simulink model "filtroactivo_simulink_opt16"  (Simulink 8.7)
settings: Solver=ode45  StartTime=0.0  StopTime=4  RelTol=1e-3
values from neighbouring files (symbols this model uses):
  C_LPF = 90e-6;5e-6;1e-6    [filtroactivo_simulink_opt16_default_values.m]    (also in filtroactivo_simulink_discrete_6_default_values.m; filtroactivo_LPF_C.m = 5.7e-06; filtroactivo_LPF_C_1.m = C; filtroactivo_LPF_C_2.m = 1.67e-05)
  Iload_dephase = 0*pi/180 * [1 0 0 0 0 0 0]    [filtroactivo_simulink_opt16_default_values.m]    (also in filtroactivo_simulink_discrete_6_default_values.m)
  Iload_freq = 50*[1 5 7 11 13 17 19]    [filtroactivo_simulink_opt16_default_values.m]    (also in filtroactivo_simulink_discrete_6_default_values.m)
  Iload_peak = 16*sqrt(2)/100*[100 10 10 10 10 0 0]    [filtroactivo_simulink_opt16_default_values.m]    (also in filtroactivo_simulink_discrete_6_default_values.m)
  Iload_sampletime = 1e-6    (= 1e-06)    [filtroactivo_simulink_opt16_default_values.m]    (also in filtroactivo_simulink_discrete_6_default_values.m)
  Iload_simetric = [-1 1 -1 1 -1 1 -1]    [filtroactivo_simulink_opt16_default_values.m]    (also in filtroactivo_simulink_discrete_6_default_values.m)
  kI_Ired_ref = 1e-3;1e-1    [filtroactivo_simulink_opt16_default_values.m]
  kP_Ired_ref = 1e-4;2.5e-4;1e-2    [filtroactivo_simulink_opt16_default_values.m]
  L_grid = 15e-6    (= 1.5e-05)    [filtroactivo_simulink_opt16_default_values.m]    (also in filtroactivo_simulink_discrete_6_default_values.m; filtroactivo_LPF_C_2.m)
  L_LPF = L    (= 0.004)    [filtroactivo_LPF_C.m]    (also in filtroactivo_LPF_C_1.m = L; filtroactivo_LPF_L.m = 0.001)
  period_SuSvSw = 1e-6    (= 1e-06)    [filtroactivo_simulink_opt16_default_values.m]    (also in filtroactivo_simulink_discrete_6_default_values.m)
  R_C_LPF = .1;.5    [filtroactivo_simulink_opt16_default_values.m]    (also in filtroactivo_simulink_discrete_6_default_values.m; filtroactivo_LPF_C.m = 0.5; filtroactivo_LPF_C_2.m = 0.5)
  R_grid = 0.02    [filtroactivo_simulink_opt16_default_values.m]    (also in filtroactivo_simulink_discrete_6_default_values.m; filtroactivo_LPF_C_2.m)
  R_L_LPF = .65;.125    [filtroactivo_simulink_opt16_default_values.m]    (also in filtroactivo_simulink_discrete_6_default_values.m; filtroactivo_LPF_C.m = 0.5)
  R_neutro_inverter_C_LPF = 1e-2;1;50;1e-2    [filtroactivo_simulink_opt16_default_values.m]    (also in filtroactivo_simulink_discrete_6_default_values.m)
  Vcc_desired = 900    [filtroactivo_simulink_opt16_default_values.m]    (also in filtroactivo_simulink_discrete_6_default_values.m)
  Vnet_dephase = 0*pi/180    (= 0)    [filtroactivo_simulink_opt16_default_values.m]    (also in filtroactivo_simulink_discrete_6_default_values.m)
  Vnet_freq = 50    [filtroactivo_simulink_opt16_default_values.m]    (also in filtroactivo_simulink_discrete_6_default_values.m)
  Vnet_peak = 566    [filtroactivo_simulink_opt16_default_values.m]    (also in filtroactivo_simulink_discrete_6_default_values.m)
libraries: powerlib x36

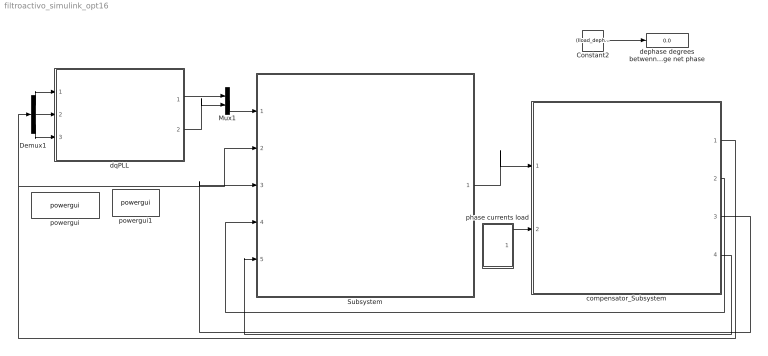
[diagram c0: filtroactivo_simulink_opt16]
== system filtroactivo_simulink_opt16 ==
  Constant2 : Constant  Value=(Iload_dephase(1) - Vnet_dephase(1))/(pi/180)
  Demux1 : Demux  Outputs=3
  Mux1 : Mux  Inputs=2
  Subsystem : Subsystem
  compensator_Subsystem : Subsystem
  dephase degrees betwenn: 1) current load phase 2) voltage net phase : Display
  dqPLL : ModelReference  ModelNameDialog=Park_method4_simulink_opt5_9_2.mdl  SimulationMode=Normal  ModelReferenceVersion=1.922
  phase currents load : Subsystem
  powergui : powerlib/powergui  Priority=1  SimulationMode=Discrete  SolverType=Tustin  SampleTime=500e-9  frequency=60  SPID=off  DisableSnubberDevices=off  DisableRonSwitches=off  DisableVfSwitches=off  SwTol=0  DisplayEquations=off  Interpol=off  ExternalGateDelay=off  methode=off  Ts=10  FunctionMessages=off  echomessages=off  HookPort=off  EnableUseOfTLC=off  x0status=blocks  frequencyindice=0  Pbase=100e6  ErrMax=1e-4  Iterations=50  UnitsV=kV  UnitsW=MW  buscounter=0  RestoreLinks=warning  ResistiveCurrentMeasurement=off  Frange=[0:2:500]  Ylog=off  Xlog=on  ShowGrid=off  save=off  variable=ZData  structure=ScopeData_compensator_Subsystem__Scope11  ZoomFFT=off  StartTime=0.5  cycles=5  DisplayStyle=1  fundamental=50  FreqAxis=on  MaxFrequency=20*50  frequencyindicesteady=1  RmsSteady=1  display=off
  powergui1 : powerlib/powergui  Priority=1  SimulationMode=Continuous  SolverType=Tustin/Backward Euler (TBE)  SampleTime=50e-6  frequency=60  SPID=off  DisableSnubberDevices=off  DisableRonSwitches=off  DisableVfSwitches=off  SwTol=0  DisplayEquations=off  Interpol=off  ExternalGateDelay=off  methode=off  Ts=10  FunctionMessages=off  echomessages=off  HookPort=off  EnableUseOfTLC=off  x0status=blocks  frequencyindice=60  Pbase=100e6  ErrMax=1e-4  Iterations=50  UnitsV=kV  UnitsW=MW  buscounter=0  RestoreLinks=warning  ResistiveCurrentMeasurement=off  Frange=[0:2:500]  Ylog=off  Xlog=on  ShowGrid=off  save=off  variable=ZData  structure=simout_I_phase_compensator_measured  ZoomFFT=off  StartTime=0.2  cycles=5  DisplayStyle=3  fundamental=50  FreqAxis=off  MaxFrequency=1000  frequencyindicesteady=1  RmsSteady=1  display=off
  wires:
  Subsystem/1(Iphase_compensator_reference) -> compensator_Subsystem/1(Iphase_compensator_reference)
  compensator_Subsystem/2(Vcc_ref-Vcc_measured) -> Subsystem/4(Vcc_ref-Vcc_measured)
  Constant2/1 -> dephase degrees betwenn: 1) current load phase 2) voltage net phase/1
  Mux1/1 -> Subsystem/1(Valpha&beta_phase_dqPLL)
  compensator_Subsystem/1(Vphase_net_measured) -> Demux1/1, Subsystem/2(Vphase_net_measured)
  compensator_Subsystem/3(Iphase_load_measured) -> Subsystem/3(I_phase_load_measured)
  compensator_Subsystem/4(Iphase_C_LPF_measured) -> Subsystem/5(Iphase_C_LPF_measured)
  phase currents load/1(Out1) -> compensator_Subsystem/2(Iphase_load_reference)
  Demux1/1 -> dqPLL/1
  Demux1/2 -> dqPLL/2
  Demux1/3 -> dqPLL/3
  dqPLL/1 -> Mux1/1
  dqPLL/2 -> Mux1/2

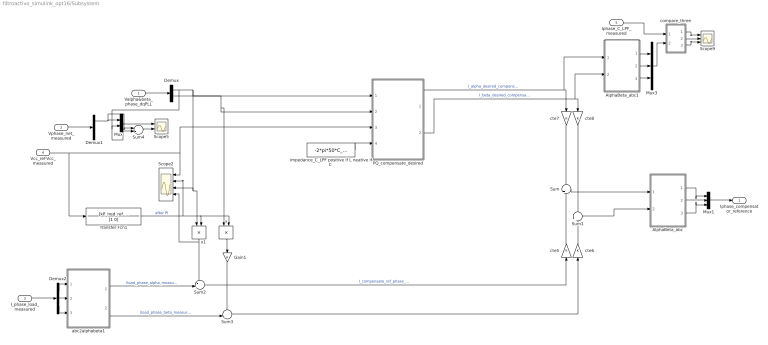
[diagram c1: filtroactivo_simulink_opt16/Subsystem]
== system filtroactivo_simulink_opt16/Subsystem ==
  Valpha&beta_phase_dqPLL : Inport
  Vphase_net_measured : Inport  Port=2
  I_phase_load_measured : Inport  Port=3
  Vcc_ref-Vcc_measured : Inport  Port=4
  Iphase_C_LPF_measured : Inport  Port=5
  AlphaBeta_abc : MATLAB Function  TreatAsAtomicUnit=on
  AlphaBeta_abc1 : MATLAB Function  TreatAsAtomicUnit=on
  Demux : Demux  Outputs=2
  Demux1 : Demux  Outputs=3
  Demux2 : Demux  Outputs=3
  Gain1 : Gain
  Mux : Mux  Inputs=2
  Mux1 : Mux  Inputs=3
  Mux3 : Mux  Inputs=3
  PQ_compensate_desired : Subsystem
  Scope2 : Scope  NumInputPorts=4
  Scope5 : Scope  NumInputPorts=2
  Scope9 : Scope  NumInputPorts=3
  Sum : Sum  Inputs=+|+
  Sum1 : Sum  Inputs=+|+
  Sum2 : Sum  Inputs=-+|
  Sum3 : Sum  Inputs=-+|
  Sum4 : Sum  Inputs=+-
  Transfer Fcn1 : TransferFcn  Numerator=[kP_Ired_ref kI_Ired_ref]  Denominator=[1 0]
  abc2alphabeta1 : MATLAB Function  TreatAsAtomicUnit=on
  compare_three : Subsystem
  cte{5..8} (4 alike) : Gain
  "impedance_C_LPF positive if L neative if C " : Constant  Value=-2*pi*50*C_LPF
  x : Product
  x1 : Product
  Iphase_compensator_reference : Outport  InitialOutput=0
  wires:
  AlphaBeta_abc/3(c) -> Mux1/3
  AlphaBeta_abc/2(b) -> Mux1/2
  AlphaBeta_abc/1(a) -> Mux1/1
  abc2alphabeta1/2(beta) -> Sum3/2  "Iload_phase_beta_measured"
  abc2alphabeta1/1(alpha) -> Sum2/2  "Iload_phase_alpha_measured"
  x/1 -> Gain1/1
  Sum/1 -> AlphaBeta_abc/1(alpha)
  Sum1/1 -> AlphaBeta_abc/2(beta)
  Sum2/1 -> cte5/1  "I_compensate_ref_phase_alpha_because_DVcc"
  Sum3/1 -> cte6/1
  cte7/1 -> Sum/1
  cte8/1 -> Sum1/1
  Vcc_ref-Vcc_measured/1 -> Transfer Fcn1/1, PQ_compensate_desired/3(Vcc_ref-Vcc_measured), Scope2/1
  Transfer Fcn1/1 -> Scope2/2, x1/2, x/2  "after PI"
  PQ_compensate_desired/2(Out2) -> AlphaBeta_abc1/2(beta), cte8/1  "I_beta_desired_compensate_PQ"
  PQ_compensate_desired/1(Out1) -> cte7/1, AlphaBeta_abc1/1(alpha)  "I_alpha_desired_compensate_PQ"
  Valpha&beta_phase_dqPLL/1 -> Demux/1
  Demux/1 -> Sum4/2, Mux/2, PQ_compensate_desired/1(Valpha), Scope2/3, x1/1
  Demux/2 -> x/1, PQ_compensate_desired/2(Vbeta)
  Vphase_net_measured/1 -> Demux1/1
  Demux1/1 -> Sum4/1, Mux/1
  Mux1/1 -> Iphase_compensator_reference/1
  Mux/1 -> Scope5/1
  Sum4/1 -> Scope5/2
  Demux2/2 -> abc2alphabeta1/2(b)
  Demux2/3 -> abc2alphabeta1/3(c)
  Demux2/1 -> abc2alphabeta1/1(a)
  cte5/1 -> Sum/2
  cte6/1 -> Sum1/2
  I_phase_load_measured/1 -> Demux2/1
  x1/1 -> Sum2/1, Scope2/4
  Gain1/1 -> Sum3/1
  "impedance_C_LPF positive if L neative if C "/1 -> PQ_compensate_desired/4(impedance_C_LPF)
  compare_three/1(Out1) -> Scope9/1
  compare_three/2(Out2) -> Scope9/2
  compare_three/3(Out3) -> Scope9/3
  Iphase_C_LPF_measured/1 -> compare_three/1(In1)
  AlphaBeta_abc1/1(a) -> Mux3/1
  AlphaBeta_abc1/2(b) -> Mux3/2
  AlphaBeta_abc1/3(c) -> Mux3/3
  Mux3/1 -> compare_three/2(In2)

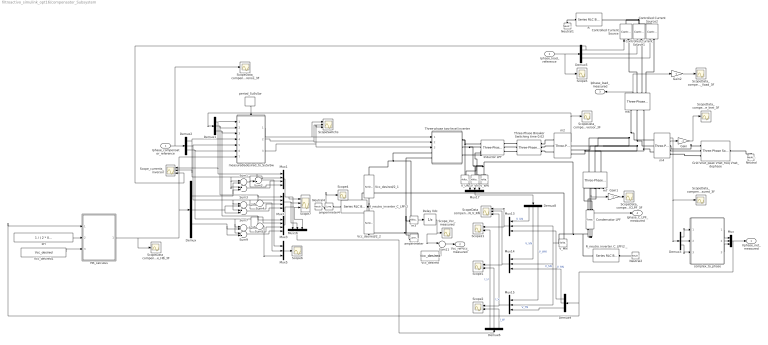
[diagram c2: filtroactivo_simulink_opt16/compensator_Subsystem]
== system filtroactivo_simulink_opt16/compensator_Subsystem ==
  Iphase_compensator_reference : Inport
  Iphase_load_reference : Inport  Port=2
  Condensator LPF : powerlib/Elements/Three-Phase Series RLC Branch  LConnTagsString=A|B|C  RConnTagsString=A|B|C  BranchType=RC  Resistance=R_C_LPF  Inductance=1e-3  Capacitance=C_LPF  Measurements=None
  Controlled Current Source : powerlib/Electrical Sources/Controlled Current Source  Initialize=off  Source_Type=AC  Amplitude=0  Phase=0  Frequency=0  Measurements=None
  Controlled Current Source1 : powerlib/Electrical Sources/Controlled Current Source  Initialize=off  Source_Type=AC  Amplitude=0  Phase=0  Frequency=0  Measurements=None
  Controlled Current Source2 : powerlib/Electrical Sources/Controlled Current Source  Initialize=off  Source_Type=AC  Amplitude=0  Phase=0  Frequency=0  Measurements=None
  Delay Vdc : UnitDelay  SampleTime=-1
  Demux{,1..3,5..6,8..9} (8 alike) : Demux  Outputs=3
  Gain : Gain  Gain=-1
  Gain1 : Gain  Gain=-1
  Gain2 : Gain  Gain=-1
  Grid Vnet_peak Vnet_freq Vnet_dephase : powerlib/Electrical Sources/Three-Phase Source  InternalConnection=Yn  VoltagePhases=off  Voltage=Vnet_peak/sqrt(2)  PhaseAngle=Vnet_dephase/pi*180  Voltage_phases=[25e3 25e3 25e3]/sqrt(3)  PhaseAngles_phases=[0 -120 +120]  Frequency=Vnet_freq  NonIdealSource=on  SpecifyImpedance=off  Resistance=R_grid  Inductance=L_grid  ShortCircuitLevel=100e6  BaseVoltage=25e3  XRratio=7  BusType=swing  Pref=0  Qref=0  Prefabc=[10e3, 10e3, 10e3]  Qrefabc=[0, 0, 0]  Qmin=-inf  Qmax=inf
  HB_calculus : MATLAB Function  TreatAsAtomicUnit=on
  Inductor LPF : powerlib/Elements/Three-Phase Series RLC Branch  LConnTagsString=A|B|C  RConnTagsString=A|B|C  BranchType=RL  Resistance=R_L_LPF  Inductance=L_LPF  Capacitance=1e-6  Measurements=None
  Mux{,5,13..17} (7 alike) : Mux  Inputs=3
  Mux1 : Mux
  Mux2 : Mux
  Mux3 : Mux
  Neutral : powerlib/Elements/Neutral  LConnTagsString=a  NodeNumber=1
  Neutral1 : powerlib/Elements/Neutral  LConnTagsString=a  NodeNumber=2
  Neutral2 : powerlib/Elements/Neutral  LConnTagsString=a  NodeNumber=2
  Neutral4 : powerlib/Elements/Neutral  LConnTagsString=a  NodeNumber=2
  R : powerlib/Elements/Series RLC Branch  LConnTagsString=__new0  RConnTagsString=__new0  BranchType=R  Resistance=1  Inductance=1e-3  SetiL0=off  InitialCurrent=0  Capacitance=1e-6  Setx0=off  InitialVoltage=0  Measurements=None
  R_neutro_inverter_C_LPF/2 : powerlib/Elements/Series RLC Branch  LConnTagsString=__new0  RConnTagsString=__new0  BranchType=R  Resistance=R_neutro_inverter_C_LPF/2  Inductance=1e-3  SetiL0=off  InitialCurrent=0  Capacitance=1e-6  Setx0=off  InitialVoltage=0  Measurements=None
  R_neutro_inverter_C_LPF/2 _ : powerlib/Elements/Series RLC Branch  LConnTagsString=__new0  RConnTagsString=__new0  BranchType=R  Resistance=R_neutro_inverter_C_LPF/2  Inductance=1e-3  SetiL0=off  InitialCurrent=0  Capacitance=1e-6  Setx0=off  InitialVoltage=0  Measurements=None
  Scope1 : Scope  NumInputPorts=2
  Scope2 : Scope  NumInputPorts=2
  Scope21 : Scope  NumInputPorts=2
  Scope4 : Scope
  Scope5 : Scope
  Scope6 : Scope
  Scope7 : Scope  NumInputPorts=3
  ScopeData_compensator_Subsystem__Scope_HB_3F : Scope
  ScopeData_compensator_Subsystem__Scope_ICLPF_3F : Scope
  ScopeData_compensator_Subsystem__Scope_Iinversor_3F : Scope
  ScopeData_compensator_Subsystem__Scope_Iinversorreference_3F : Scope
  ScopeData_compensator_Subsystem__Scope_Iload_3F : Scope
  ScopeData_compensator_Subsystem__Scope_Inet_3F : Scope
  ScopeData_compensator_Subsystem__Scope_V_UN_V_MN_V_RN : Scope  NumInputPorts=3
  ScopeData_compensator_Subsystem__Scope_Vnet_measured_3F : Scope
  ScopeSwitchs : Scope  NumInputPorts=3
  Scope_Vcc_measured : Scope
  Scope_currents_inversor : Scope  NumInputPorts=3
  Sum1 : Sum  Inputs=+-
  Sum11 : Sum  Inputs=|-+
  Sum2 : Sum  Inputs=-+|
  Sum3 : Sum
  Sum4 : Sum  Inputs=-+|
  Sum5 : Sum  Inputs=-+|
  Sum6 : Sum  Inputs=+-
  Sum7 : Sum
  Sum8 : Sum  Inputs=+-
  Sum9 : Sum
  Three-Phase Breaker Switching time 0.02 : powerlib/Elements/Three-Phase Breaker  InitialState=open  SwitchA=on  SwitchB=on  SwitchC=on  SwitchTimes=[0.020]  External=off  BreakerResistance=0.001  SnubberResistance=1e6  SnubberCapacitance=inf  Measurements=None
  Three-phase two-level inverter : Subsystem
  V_MN : powerlib/Measurements/Voltage Measurement  PhasorSimulation=off  OutputType=Complex  PSBequivalent=0
  V_UN : powerlib/Measurements/Voltage Measurement  PhasorSimulation=off  OutputType=Complex  PSBequivalent=0
  V_VN : powerlib/Measurements/Voltage Measurement  PhasorSimulation=off  OutputType=Complex  PSBequivalent=0
  V_WN : powerlib/Measurements/Voltage Measurement  PhasorSimulation=off  OutputType=Complex  PSBequivalent=0
  Vcc_desired : Constant  Value=Vcc_desired
  Vcc_desired/2_1 : powerlib/Elements/Series RLC Branch  LConnTagsString=__new0  RConnTagsString=__new0  BranchType=C  Resistance=0  Inductance=0  SetiL0=off  InitialCurrent=0  Capacitance=1e-2  Setx0=on  InitialVoltage=Vcc_desired/2  Measurements=None
  Vcc_desired/2_2 : powerlib/Elements/Series RLC Branch  LConnTagsString=__new0  RConnTagsString=__new0  BranchType=C  Resistance=0  Inductance=0  SetiL0=off  InitialCurrent=0  Capacitance=1e-2  Setx0=on  InitialVoltage=Vcc_desired/2  Measurements=None
  Vcc_desired1 : Constant  Value=Vcc_desired
  amperimeter : powerlib/Measurements/Current Measurement  PhasorSimulation=off  OutputType=Complex  PSBequivalent=0
  amperimeter4 : powerlib/Measurements/Current Measurement  PhasorSimulation=off  OutputType=Complex  PSBequivalent=0
  complex_to_phase : MATLAB Function  TreatAsAtomicUnit=on
  kH : Constant  Value=1 / ( 2 * 0.005 * 25e3 *Vcc_desired )
  m{2,4,6..7} (4 alike) : powerlib/Measurements/Three-Phase V-I Measurement  VoltageMeasurement=phase-to-phase  SetLabelV=off  LabelV=Vabc  Vpu=off  VpuLL=off  CurrentMeasurement=yes  SetLabelI=off  LabelI=Iabc  Ipu=off  Pbase=100e6  Vbase=500e3  OutputType=Complex  PhasorSimulation=off  PSBequivalent=0
  m3 : powerlib/Measurements/Voltage Measurement  PhasorSimulation=off  OutputType=Complex  PSBequivalent=0
  measured&desired_to_SuSvSw : Subsystem
  period_SuSvSw : DiscretePulseGenerator  PulseType=Time based  Period=period_SuSvSw  PulseWidth=50
  Vphase_net_measured : Outport
  Vcc_ref-Vcc_measured : Outport  Port=2
  Iphase_load_measured : Outport  Port=3
  Iphase_C_LPF_measured : Outport  Port=4
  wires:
  period_SuSvSw/1 -> measured&desired_to_SuSvSw/Trigger
  Demux2/1 -> measured&desired_to_SuSvSw/4(Iu*), Sum2/2, Mux1/2, Sum1/1, Sum3/1, Scope_currents_inversor/2
  Demux2/2 -> measured&desired_to_SuSvSw/5(Iv*), Sum7/1, Sum6/1, Mux2/2, Sum4/2
  Demux2/3 -> measured&desired_to_SuSvSw/6(Iw*), Sum9/1, Sum8/1, Mux3/2, Sum5/2
  Sum1/1 -> Mux1/4
  Sum3/1 -> Mux1/3
  Sum6/1 -> Mux2/3
  Sum8/1 -> Mux3/3
  Demux/1 -> Sum1/2, Sum3/2
  Demux/2 -> Sum6/2, Sum7/2
  Demux/3 -> Sum9/2, Sum8/2
  m3/1 -> Delay Vdc/1
  Delay Vdc/1 -> Sum11/1, Scope_Vcc_measured/1
  HB_calculus/1(HB) -> ScopeData_compensator_Subsystem__Scope_HB_3F/1, Demux/1, measured&desired_to_SuSvSw/7(H)
  m4/1 -> ScopeData_compensator_Subsystem__Scope_Vnet_measured_3F/1, Demux3/1
  m4/2 -> Gain/1
  Demux1/2 -> Sum4/1, Mux2/1, measured&desired_to_SuSvSw/2(Iv)
  Demux1/3 -> measured&desired_to_SuSvSw/3(Iw), Sum5/1, Mux3/1
  Demux1/1 -> Scope_currents_inversor/1, Sum2/1, Mux1/1, measured&desired_to_SuSvSw/1(Iu)
  Demux5/1 -> Scope_currents_inversor/3, Controlled Current Source/1
  Demux5/2 -> Controlled Current Source1/1
  Demux5/3 -> Controlled Current Source2/1
  m7/2 -> Gain1/1, Iphase_C_LPF_measured/1
  Iphase_load_reference/1 -> Scope5/1, Demux5/1
  m6/2 -> Gain2/1, Iphase_load_measured/1
  Mux5/1 -> Scope6/1
  Sum2/1 -> Mux5/1
  Sum4/1 -> Mux5/2
  Sum5/1 -> Mux5/3
  Sum7/1 -> Mux2/4
  Sum9/1 -> Mux3/4
  Gain/1 -> ScopeData_compensator_Subsystem__Scope_Inet_3F/1
  m2/2 -> ScopeData_compensator_Subsystem__Scope_Iinversor_3F/1, Demux1/1
  Sum11/1 -> Vcc_ref-Vcc_measured/1
  Vcc_desired/1 -> Sum11/2
  Demux3/2 -> complex_to_phase/2(Vst)
  Demux3/1 -> complex_to_phase/1(Vrs)
  Demux3/3 -> complex_to_phase/3(Vtr)
  complex_to_phase/2(Vs) -> Mux/2
  complex_to_phase/3(Vt) -> Mux/3
  complex_to_phase/1(Vr) -> Mux/1
  Iphase_compensator_reference/1 -> ScopeData_compensator_Subsystem__Scope_Iinversorreference_3F/1, Demux2/1
  amperimeter4/1 -> Scope4/1
  measured&desired_to_SuSvSw/3(Sw) -> Three-phase two-level inverter/3(Sc), ScopeSwitchs/3
  measured&desired_to_SuSvSw/2(Sv) -> ScopeSwitchs/2, Three-phase two-level inverter/2(Sb)
  measured&desired_to_SuSvSw/1(Su) -> ScopeSwitchs/1, Three-phase two-level inverter/1(Sa)
  Mux/1 -> Demux9/1, HB_calculus/1(Vfaseneutro), Vphase_net_measured/1
  kH/1 -> HB_calculus/2(Kh)
  Vcc_desired1/1 -> HB_calculus/3(Vcc_desired)
  Gain1/1 -> ScopeData_compensator_Subsystem__Scope_ICLPF_3F/1
  V_VN/1 -> Mux17/2
  V_WN/1 -> Mux17/3
  V_UN/1 -> Mux17/1
  Mux13/1 -> Scope21/1, ScopeData_compensator_Subsystem__Scope_V_UN_V_MN_V_RN/1
  Mux14/1 -> Scope1/1, ScopeData_compensator_Subsystem__Scope_V_UN_V_MN_V_RN/2
  V_MN/1 -> Mux15/2, Mux14/2, Mux13/2
  Demux8/1 -> Mux13/1  "V_UN"
  Demux8/2 -> Mux14/1  "V_VN"
  Demux8/3 -> Mux15/1  "V_WN"
  Demux9/1 -> Mux13/3  "V_RN"
  Demux9/2 -> Mux14/3  "V_SN"
  Demux9/3 -> Mux15/3  "V_TN"
  Mux15/1 -> Scope2/1, ScopeData_compensator_Subsystem__Scope_V_UN_V_MN_V_RN/3
  Mux17/1 -> Demux8/1
  Mux1/1 -> Mux16/1, Scope7/1
  Mux2/1 -> Mux16/2, Scope7/2
  Mux3/1 -> Mux16/3, Scope7/3
  Mux16/1 -> Demux6/1
  Demux6/1 -> Scope21/2  "I_U"
  Demux6/2 -> Scope1/2  "I_V"
  Demux6/3 -> Scope2/2  "I_W"
  Gain2/1 -> ScopeData_compensator_Subsystem__Scope_Iload_3F/1
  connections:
  Three-phase two-level inverter/RConn1 -- V_UN/LConn1 -- Inductor LPF/LConn1
  Three-phase two-level inverter/RConn2 -- V_VN/LConn1 -- Inductor LPF/LConn2
  Vcc_desired/2_2/RConn1 -- m3/LConn2 -- amperimeter/LConn1
  Three-phase two-level inverter/LConn1 -- Vcc_desired/2_1/LConn1 -- m3/LConn1
  m6/LConn1 -- m7/LConn1 -- m2/RConn1 -- m4/LConn1
  Controlled Current Source1/RConn1 -- R/RConn1 -- Controlled Current Source/RConn1 -- Controlled Current Source2/RConn1
  m6/LConn2 -- m7/LConn2 -- m2/RConn2 -- m4/LConn2
  m6/LConn3 -- m7/LConn3 -- m2/RConn3 -- m4/LConn3
  m6/RConn1 -- Controlled Current Source/LConn1
  Neutral1/LConn1 -- R/LConn1
  m4/RConn2 -- Grid Vnet_peak Vnet_freq Vnet_dephase/RConn2
  Grid Vnet_peak Vnet_freq Vnet_dephase/LConn1 -- Neutral/LConn1
  Condensator LPF/LConn1 -- m7/RConn1
  m4/RConn1 -- Grid Vnet_peak Vnet_freq Vnet_dephase/RConn1
  Condensator LPF/LConn3 -- m7/RConn3
  Three-Phase Breaker Switching time 0.02/RConn1 -- m2/LConn1
  Condensator LPF/LConn2 -- m7/RConn2
  m6/RConn2 -- Controlled Current Source1/LConn1
  amperimeter/RConn1 -- Three-phase two-level inverter/LConn2
  Three-Phase Breaker Switching time 0.02/RConn3 -- m2/LConn3
  Three-Phase Breaker Switching time 0.02/RConn2 -- m2/LConn2
  m6/RConn3 -- Controlled Current Source2/LConn1
  R_neutro_inverter_C_LPF/2 _/LConn1 -- Neutral2/LConn1
  Inductor LPF/LConn3 -- V_WN/LConn1 -- Three-phase two-level inverter/RConn3
  m4/RConn3 -- Grid Vnet_peak Vnet_freq Vnet_dephase/RConn3
  R_neutro_inverter_C_LPF/2/RConn1 -- V_MN/LConn1 -- Vcc_desired/2_1/RConn1 -- Vcc_desired/2_2/LConn1
  amperimeter4/LConn1 -- Neutral4/LConn1
  amperimeter4/RConn1 -- R_neutro_inverter_C_LPF/2/LConn1
  Inductor LPF/RConn1 -- Three-Phase Breaker Switching time 0.02/LConn1
  Inductor LPF/RConn2 -- Three-Phase Breaker Switching time 0.02/LConn2
  Inductor LPF/RConn3 -- Three-Phase Breaker Switching time 0.02/LConn3
  Condensator LPF/RConn1 -- V_VN/LConn2 -- V_UN/LConn2 -- V_WN/LConn2 -- V_MN/LConn2 -- R_neutro_inverter_C_LPF/2 _/RConn1 -- Condensator LPF/RConn3 -- Condensator LPF/RConn2

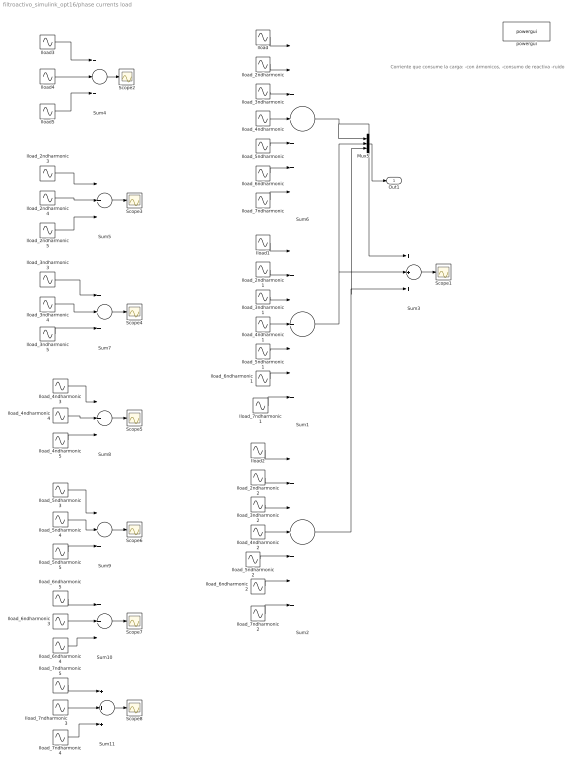
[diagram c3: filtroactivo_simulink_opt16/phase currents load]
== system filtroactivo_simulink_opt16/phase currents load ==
  note: Corriente que consume la carga: -con ármonicos, -consumo de reactiva -ruido
  Iload : Sin  Amplitude=Iload_peak(1)  Frequency=2*pi*Iload_freq(1)  Phase=Iload_dephase(1)  SampleTime=Iload_sampletime
  Iload1 : Sin  Amplitude=Iload_peak(1)  Frequency=2*pi*Iload_freq(1)  Phase=Iload_dephase(1) + 2*pi/3*Iload_simetric(1)  SampleTime=Iload_sampletime
  Iload2 : Sin  Amplitude=Iload_peak(1)  Frequency=2*pi*Iload_freq(1)  Phase=Iload_dephase(1) + 4*pi/3*Iload_simetric(1)  SampleTime=Iload_sampletime
  Iload3 : Sin  Amplitude=Iload_peak(1)  Frequency=2*pi*Iload_freq(1)  Phase=Iload_dephase(1)  SampleTime=Iload_sampletime
  Iload4 : Sin  Amplitude=Iload_peak(1)  Frequency=2*pi*Iload_freq(1)  Phase=Iload_dephase(1) + 2*pi/3*Iload_simetric(1)  SampleTime=Iload_sampletime
  Iload5 : Sin  Amplitude=Iload_peak(1)  Frequency=2*pi*Iload_freq(1)  Phase=Iload_dephase(1) + 4*pi/3*Iload_simetric(1)  SampleTime=Iload_sampletime
  Iload_2ndharmonic : Sin  Amplitude=Iload_peak(2)  Frequency=2*pi*Iload_freq(2)  Phase=Iload_dephase(2)  SampleTime=Iload_sampletime
  Iload_2ndharmonic1 : Sin  Amplitude=Iload_peak(2)  Frequency=2*pi*Iload_freq(2)  Phase=Iload_dephase(2) + 2*pi/3*Iload_simetric(2)  SampleTime=Iload_sampletime
  Iload_2ndharmonic2 : Sin  Amplitude=Iload_peak(2)  Frequency=2*pi*Iload_freq(2)  Phase=Iload_dephase(2) + 4*pi/3*Iload_simetric(2)  SampleTime=Iload_sampletime
  Iload_2ndharmonic3 : Sin  Amplitude=Iload_peak(2)  Frequency=2*pi*Iload_freq(2)  Phase=Iload_dephase(2)  SampleTime=Iload_sampletime
  Iload_2ndharmonic4 : Sin  Amplitude=Iload_peak(2)  Frequency=2*pi*Iload_freq(2)  Phase=Iload_dephase(2) + 2*pi/3*Iload_simetric(2)  SampleTime=Iload_sampletime
  Iload_2ndharmonic5 : Sin  Amplitude=Iload_peak(2)  Frequency=2*pi*Iload_freq(2)  Phase=Iload_dephase(2) + 4*pi/3*Iload_simetric(2)  SampleTime=Iload_sampletime
  Iload_3ndharmonic : Sin  Amplitude=Iload_peak(3)  Frequency=2*pi*Iload_freq(3)  Phase=Iload_dephase(3)  SampleTime=Iload_sampletime
  Iload_3ndharmonic1 : Sin  Amplitude=Iload_peak(3)  Frequency=2*pi*Iload_freq(3)  Phase=Iload_dephase(3) + 2*pi/3*Iload_simetric(3)  SampleTime=Iload_sampletime
  Iload_3ndharmonic2 : Sin  Amplitude=Iload_peak(3)  Frequency=2*pi*Iload_freq(3)  Phase=Iload_dephase(3) + 4*pi/3*Iload_simetric(3)  SampleTime=Iload_sampletime
  Iload_3ndharmonic3 : Sin  Amplitude=Iload_peak(3)  Frequency=2*pi*Iload_freq(3)  Phase=Iload_dephase(3)  SampleTime=Iload_sampletime
  Iload_3ndharmonic4 : Sin  Amplitude=Iload_peak(3)  Frequency=2*pi*Iload_freq(3)  Phase=Iload_dephase(3) + 2*pi/3*Iload_simetric(3)  SampleTime=Iload_sampletime
  Iload_3ndharmonic5 : Sin  Amplitude=Iload_peak(3)  Frequency=2*pi*Iload_freq(3)  Phase=Iload_dephase(3) + 4*pi/3*Iload_simetric(3)  SampleTime=Iload_sampletime
  Iload_4ndharmonic : Sin  Amplitude=Iload_peak(4)  Frequency=2*pi*Iload_freq(4)  Phase=Iload_dephase(4)  SampleTime=Iload_sampletime
  Iload_4ndharmonic1 : Sin  Amplitude=Iload_peak(4)  Frequency=2*pi*Iload_freq(4)  Phase=Iload_dephase(4) + 2*pi/3*Iload_simetric(4)  SampleTime=Iload_sampletime
  Iload_4ndharmonic2 : Sin  Amplitude=Iload_peak(4)  Frequency=2*pi*Iload_freq(4)  Phase=Iload_dephase(4) + 4*pi/3*Iload_simetric(4)  SampleTime=Iload_sampletime
  Iload_4ndharmonic3 : Sin  Amplitude=Iload_peak(4)  Frequency=2*pi*Iload_freq(4)  Phase=Iload_dephase(4)  SampleTime=Iload_sampletime
  Iload_4ndharmonic4 : Sin  Amplitude=Iload_peak(4)  Frequency=2*pi*Iload_freq(4)  Phase=Iload_dephase(4) + 2*pi/3*Iload_simetric(4)  SampleTime=Iload_sampletime
  Iload_4ndharmonic5 : Sin  Amplitude=Iload_peak(4)  Frequency=2*pi*Iload_freq(4)  Phase=Iload_dephase(4) + 4*pi/3*Iload_simetric(4)  SampleTime=Iload_sampletime
  Iload_5ndharmonic : Sin  Amplitude=Iload_peak(5)  Frequency=2*pi*Iload_freq(5)  Phase=Iload_dephase(5)  SampleTime=Iload_sampletime
  Iload_5ndharmonic1 : Sin  Amplitude=Iload_peak(5)  Frequency=2*pi*Iload_freq(5)  Phase=Iload_dephase(5) + 2*pi/3*Iload_simetric(5)  SampleTime=Iload_sampletime
  Iload_5ndharmonic2 : Sin  Amplitude=Iload_peak(5)  Frequency=2*pi*Iload_freq(5)  Phase=Iload_dephase(5) + 4*pi/3*Iload_simetric(5)  SampleTime=Iload_sampletime
  Iload_5ndharmonic3 : Sin  Amplitude=Iload_peak(5)  Frequency=2*pi*Iload_freq(5)  Phase=Iload_dephase(5)  SampleTime=Iload_sampletime
  Iload_5ndharmonic4 : Sin  Amplitude=Iload_peak(5)  Frequency=2*pi*Iload_freq(5)  Phase=Iload_dephase(5) + 2*pi/3*Iload_simetric(5)  SampleTime=Iload_sampletime
  Iload_5ndharmonic5 : Sin  Amplitude=Iload_peak(5)  Frequency=2*pi*Iload_freq(5)  Phase=Iload_dephase(5) + 4*pi/3*Iload_simetric(5)  SampleTime=Iload_sampletime
  Iload_6ndharmonic : Sin  Amplitude=Iload_peak(6)  Frequency=2*pi*Iload_freq(6)  Phase=Iload_dephase(6)  SampleTime=Iload_sampletime
  Iload_6ndharmonic1 : Sin  Amplitude=Iload_peak(6)  Frequency=2*pi*Iload_freq(6)  Phase=Iload_dephase(6) + 2*pi/3*Iload_simetric(6)  SampleTime=Iload_sampletime
  Iload_6ndharmonic2 : Sin  Amplitude=Iload_peak(6)  Frequency=2*pi*Iload_freq(6)  Phase=Iload_dephase(6) + 4*pi/3*Iload_simetric(6)  SampleTime=Iload_sampletime
  Iload_6ndharmonic3 : Sin  Amplitude=Iload_peak(6)  Frequency=2*pi*Iload_freq(6)  Phase=Iload_dephase(6) + 2*pi/3*Iload_simetric(6)  SampleTime=Iload_sampletime
  Iload_6ndharmonic4 : Sin  Amplitude=Iload_peak(6)  Frequency=2*pi*Iload_freq(6)  Phase=Iload_dephase(6) + 4*pi/3*Iload_simetric(6)  SampleTime=Iload_sampletime
  Iload_6ndharmonic5 : Sin  Amplitude=Iload_peak(6)  Frequency=2*pi*Iload_freq(6)  Phase=Iload_dephase(6)  SampleTime=Iload_sampletime
  Iload_7ndharmonic : Sin  Amplitude=Iload_peak(7)  Frequency=2*pi*Iload_freq(7)  Phase=Iload_dephase(7)  SampleTime=Iload_sampletime
  Iload_7ndharmonic1 : Sin  Amplitude=Iload_peak(7)  Frequency=2*pi*Iload_freq(7)  Phase=Iload_dephase(7) + 2*pi/3*Iload_simetric(7)  SampleTime=Iload_sampletime
  Iload_7ndharmonic2 : Sin  Amplitude=Iload_peak(7)  Frequency=2*pi*Iload_freq(7)  Phase=Iload_dephase(7) + 4*pi/3*Iload_simetric(7)  SampleTime=Iload_sampletime
  Iload_7ndharmonic3 : Sin  Amplitude=Iload_peak(7)  Frequency=2*pi*Iload_freq(7)  Phase=Iload_dephase(7) + 2*pi/3*Iload_simetric(7)  SampleTime=Iload_sampletime
  Iload_7ndharmonic4 : Sin  Amplitude=Iload_peak(7)  Frequency=2*pi*Iload_freq(7)  Phase=Iload_dephase(7) + 4*pi/3*Iload_simetric(7)  SampleTime=Iload_sampletime
  Iload_7ndharmonic5 : Sin  Amplitude=Iload_peak(7)  Frequency=2*pi*Iload_freq(7)  Phase=Iload_dephase(7)  SampleTime=Iload_sampletime
  Mux5 : Mux  Inputs=3
  Scope{1..8} (8 alike) : Scope
  Sum1 : Sum  Inputs=+++++++
  Sum{3..5,7..11} (8 alike) : Sum  Inputs=+++
  Sum2 : Sum  Inputs=+++++++
  Sum6 : Sum  Inputs=+++++++
  powergui : powerlib/powergui  Priority=1  SimulationMode=Discrete  SolverType=Tustin  SampleTime=500e-9  frequency=60  SPID=off  DisableSnubberDevices=off  DisableRonSwitches=off  DisableVfSwitches=off  SwTol=0  DisplayEquations=off  Interpol=off  ExternalGateDelay=off  methode=off  Ts=10  FunctionMessages=off  echomessages=off  HookPort=off  EnableUseOfTLC=off  x0status=blocks  frequencyindice=0  Pbase=100e6  ErrMax=1e-4  Iterations=50  UnitsV=kV  UnitsW=MW  buscounter=0  RestoreLinks=warning  ResistiveCurrentMeasurement=off  Frange=[0:2:500]  Ylog=off  Xlog=on  ShowGrid=off  save=off  variable=ZData  structure=ScopeData_compensator_Subsystem__Scope10  ZoomFFT=off  StartTime=0.14  cycles=2  DisplayStyle=3  fundamental=50  FreqAxis=on  MaxFrequency=1e3  frequencyindicesteady=1  RmsSteady=1  display=off
  Out1 : Outport
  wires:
  Mux5/1 -> Out1/1
  Iload2/1 -> Sum2/1
  Iload_2ndharmonic2/1 -> Sum2/2
  Iload_6ndharmonic2/1 -> Sum2/6
  Iload_4ndharmonic2/1 -> Sum2/4
  Iload_7ndharmonic2/1 -> Sum2/7
  Iload_5ndharmonic2/1 -> Sum2/5
  Iload_3ndharmonic2/1 -> Sum2/3
  Iload1/1 -> Sum1/1
  Iload_2ndharmonic1/1 -> Sum1/2
  Iload_6ndharmonic1/1 -> Sum1/6
  Iload_5ndharmonic1/1 -> Sum1/5
  Iload_3ndharmonic1/1 -> Sum1/3
  Iload_7ndharmonic1/1 -> Sum1/7
  Iload_4ndharmonic1/1 -> Sum1/4
  Iload/1 -> Sum6/1
  Iload_2ndharmonic/1 -> Sum6/2
  Iload_5ndharmonic/1 -> Sum6/5
  Iload_7ndharmonic/1 -> Sum6/7
  Iload_3ndharmonic/1 -> Sum6/3
  Iload_6ndharmonic/1 -> Sum6/6
  Iload_4ndharmonic/1 -> Sum6/4
  Sum6/1 -> Mux5/1, Sum3/1
  Sum1/1 -> Mux5/2, Sum3/2
  Sum2/1 -> Sum3/3, Mux5/3
  Sum3/1 -> Scope1/1
  Sum4/1 -> Scope2/1
  Sum5/1 -> Scope3/1
  Sum7/1 -> Scope4/1
  Sum8/1 -> Scope5/1
  Sum9/1 -> Scope6/1
  Sum10/1 -> Scope7/1
  Iload4/1 -> Sum4/2
  Iload3/1 -> Sum4/1
  Iload5/1 -> Sum4/3
  Iload_2ndharmonic4/1 -> Sum5/2
  Iload_2ndharmonic3/1 -> Sum5/1
  Iload_2ndharmonic5/1 -> Sum5/3
  Iload_3ndharmonic5/1 -> Sum7/3
  Iload_3ndharmonic4/1 -> Sum7/2
  Iload_3ndharmonic3/1 -> Sum7/1
  Iload_4ndharmonic5/1 -> Sum8/3
  Iload_4ndharmonic4/1 -> Sum8/2
  Iload_4ndharmonic3/1 -> Sum8/1
  Iload_5ndharmonic5/1 -> Sum9/3
  Iload_5ndharmonic4/1 -> Sum9/2
  Iload_5ndharmonic3/1 -> Sum9/1
  Sum11/1 -> Scope8/1
  Iload_7ndharmonic3/1 -> Sum11/2
  Iload_7ndharmonic5/1 -> Sum11/1
  Iload_7ndharmonic4/1 -> Sum11/3
  Iload_6ndharmonic3/1 -> Sum10/2
  Iload_6ndharmonic5/1 -> Sum10/1
  Iload_6ndharmonic4/1 -> Sum10/3

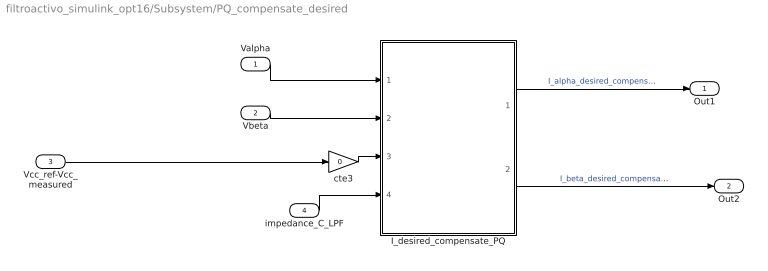
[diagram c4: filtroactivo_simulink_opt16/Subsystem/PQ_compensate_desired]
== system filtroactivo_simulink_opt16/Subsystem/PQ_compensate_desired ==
  Valpha : Inport
  Vbeta : Inport  Port=2
  Vcc_ref-Vcc_measured : Inport  Port=3
  impedance_C_LPF : Inport  Port=4
  I_desired_compensate_PQ : MATLAB Function  TreatAsAtomicUnit=on
  cte3 : Gain  Gain=0
  Out1 : Outport
  Out2 : Outport  Port=2
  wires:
  Vcc_ref-Vcc_measured/1 -> cte3/1
  I_desired_compensate_PQ/1(Ialpha) -> Out1/1  "I_alpha_desired_compensate_PQ"
  I_desired_compensate_PQ/2(Ibeta) -> Out2/1  "I_beta_desired_compensate_PQ"
  cte3/1 -> I_desired_compensate_PQ/3(Gp)
  impedance_C_LPF/1 -> I_desired_compensate_PQ/4(Gq)
  Valpha/1 -> I_desired_compensate_PQ/1(Valpha)
  Vbeta/1 -> I_desired_compensate_PQ/2(Vbeta)

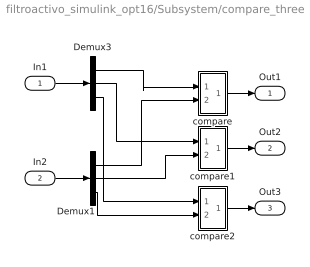
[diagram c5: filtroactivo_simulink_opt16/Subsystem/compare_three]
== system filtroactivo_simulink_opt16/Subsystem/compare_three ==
  In1 : Inport
  In2 : Inport  Port=2
  Demux1 : Demux  Outputs=3
  Demux3 : Demux  Outputs=3
  compare : Subsystem
  compare1 : Subsystem
  compare2 : Subsystem
  Out1 : Outport
  Out2 : Outport  Port=2
  Out3 : Outport  Port=3
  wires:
  In1/1 -> Demux3/1
  In2/1 -> Demux1/1
  Demux3/1 -> compare/1(In1)
  Demux1/1 -> compare/2(In2)
  Demux3/2 -> compare1/1(In1)
  Demux1/2 -> compare1/2(In2)
  Demux3/3 -> compare2/1(In1)
  Demux1/3 -> compare2/2(In2)
  compare2/1(Out1) -> Out3/1
  compare1/1(Out1) -> Out2/1
  compare/1(Out1) -> Out1/1

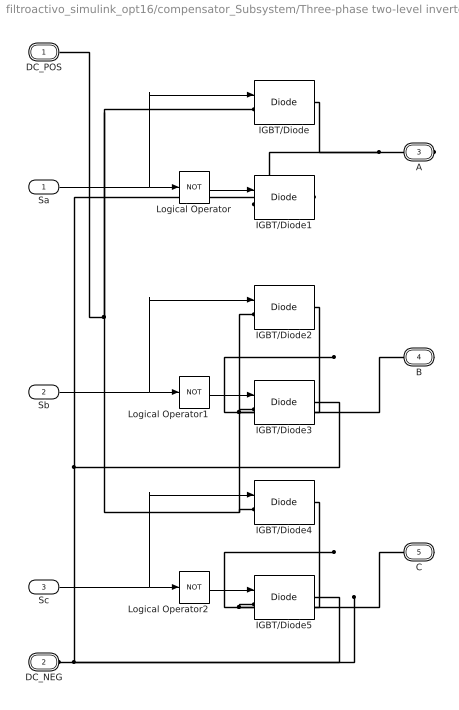
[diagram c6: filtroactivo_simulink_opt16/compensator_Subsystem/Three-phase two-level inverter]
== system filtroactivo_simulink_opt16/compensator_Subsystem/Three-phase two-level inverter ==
  Sa : Inport
  Sb : Inport  Port=2
  Sc : Inport  Port=3
  IGBT/Diode{,1..5} (6 alike) : powerlib/Power Electronics/IGBT//Diode  Ron=1e-3  Rs=1e5  Cs=inf  Measurements=off
  Logical Operator : Logic  Operator=NOT  AllPortsSameDT=off  OutDataTypeStr=boolean
  Logical Operator1 : Logic  Operator=NOT  AllPortsSameDT=off  OutDataTypeStr=boolean
  Logical Operator2 : Logic  Operator=NOT  AllPortsSameDT=off  OutDataTypeStr=boolean
  DC_POS : PMIOPort  Tag=PMCPort  Port=1  Side=Left
  DC_NEG : PMIOPort  Tag=PMCPort  Port=2  Side=Left
  A : PMIOPort  Tag=PMCPort  Port=3  Side=Right
  B : PMIOPort  Tag=PMCPort  Port=4  Side=Right
  C : PMIOPort  Tag=PMCPort  Port=5  Side=Right
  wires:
  Sc/1 -> Logical Operator2/1, IGBT/Diode4/1
  Logical Operator2/1 -> IGBT/Diode5/1
  Sb/1 -> Logical Operator1/1, IGBT/Diode2/1
  Logical Operator1/1 -> IGBT/Diode3/1
  Sa/1 -> Logical Operator/1, IGBT/Diode/1
  Logical Operator/1 -> IGBT/Diode1/1
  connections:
  IGBT/Diode5/LConn1 -- IGBT/Diode4/RConn1 -- C/RConn1
  IGBT/Diode3/LConn1 -- B/RConn1 -- IGBT/Diode2/RConn1
  IGBT/Diode4/LConn1 -- IGBT/Diode2/LConn1 -- IGBT/Diode/LConn1 -- DC_POS/RConn1
  A/RConn1 -- IGBT/Diode1/LConn1 -- IGBT/Diode/RConn1
  DC_NEG/RConn1 -- IGBT/Diode5/RConn1 -- IGBT/Diode3/RConn1 -- IGBT/Diode1/RConn1

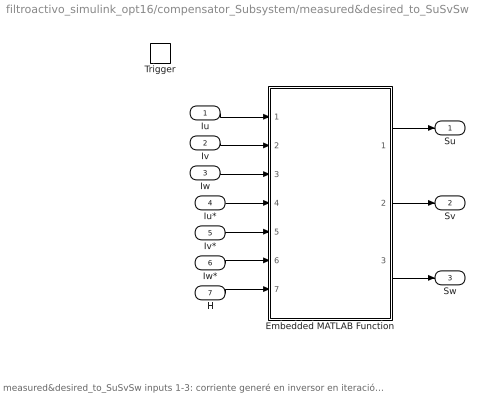
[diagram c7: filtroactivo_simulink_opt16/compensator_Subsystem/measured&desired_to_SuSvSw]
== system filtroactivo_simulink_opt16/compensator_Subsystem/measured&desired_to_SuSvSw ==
  note: measured&desired_to_SuSvSw inputs 1-3: corriente generé en inversor en iteración anterior inputs 4-6: corriente q deseo generar en inversor outputs: disparos Su,Sv,Sw q definen la corriente mas parecida a deseada que puedo generar
  Iu : Inport
  Iv : Inport  Port=2
  Iw : Inport  Port=3
  Iu* : Inport  Port=4
  Iv* : Inport  Port=5
  Iw* : Inport  Port=6
  H : Inport  Port=7
  Trigger : TriggerPort  VariantControl=Variant
  Embedded MATLAB Function : MATLAB Function  TreatAsAtomicUnit=on
  Su : Outport
  Sv : Outport  Port=2
  Sw : Outport  Port=3
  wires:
  Embedded MATLAB Function/3(Sw) -> Sw/1
  Embedded MATLAB Function/2(Sv) -> Sv/1
  Embedded MATLAB Function/1(Su) -> Su/1
  Iu/1 -> Embedded MATLAB Function/1(Iu)
  Iv/1 -> Embedded MATLAB Function/2(Iv)
  Iw/1 -> Embedded MATLAB Function/3(Iw)
  Iu*/1 -> Embedded MATLAB Function/4(Iu1)
  Iv*/1 -> Embedded MATLAB Function/5(Iv1)
  Iw*/1 -> Embedded MATLAB Function/6(Iw1)
  H/1 -> Embedded MATLAB Function/7(H)

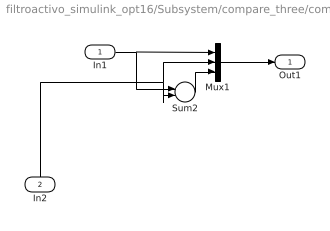
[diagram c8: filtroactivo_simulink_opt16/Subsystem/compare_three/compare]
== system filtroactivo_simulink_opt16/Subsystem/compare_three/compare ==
  In1 : Inport
  In2 : Inport  Port=2
  Mux1 : Mux  Inputs=3
  Sum2 : Sum  Inputs=+-
  Out1 : Outport
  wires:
  Sum2/1 -> Mux1/3
  Mux1/1 -> Out1/1
  In1/1 -> Sum2/1, Mux1/1
  In2/1 -> Sum2/2, Mux1/2

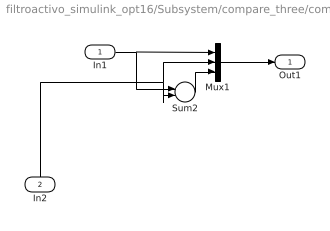
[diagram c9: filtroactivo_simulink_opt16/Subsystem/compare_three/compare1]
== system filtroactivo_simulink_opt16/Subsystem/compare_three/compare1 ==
  In1 : Inport
  In2 : Inport  Port=2
  Mux1 : Mux  Inputs=3
  Sum2 : Sum  Inputs=+-
  Out1 : Outport
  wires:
  Sum2/1 -> Mux1/3
  Mux1/1 -> Out1/1
  In1/1 -> Sum2/1, Mux1/1
  In2/1 -> Sum2/2, Mux1/2

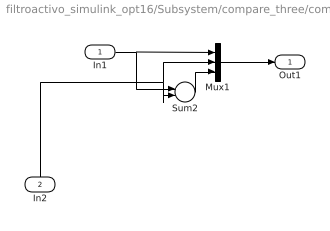
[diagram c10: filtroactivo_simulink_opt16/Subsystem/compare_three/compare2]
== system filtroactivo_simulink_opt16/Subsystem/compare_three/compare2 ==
  In1 : Inport
  In2 : Inport  Port=2
  Mux1 : Mux  Inputs=3
  Sum2 : Sum  Inputs=+-
  Out1 : Outport
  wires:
  Sum2/1 -> Mux1/3
  Mux1/1 -> Out1/1
  In1/1 -> Sum2/1, Mux1/1
  In2/1 -> Sum2/2, Mux1/2

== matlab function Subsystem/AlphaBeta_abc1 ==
function [a, b, c] = AlphaBeta_abc(alpha, beta)


a = alpha;
b = -.5 * alpha + .866 * beta;
c = -.5 * alpha - .866 * beta;

    
return

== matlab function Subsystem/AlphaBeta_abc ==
function [a, b, c] = AlphaBeta_abc(alpha, beta)


a = alpha;
b = -.5 * alpha + .866 * beta;
c = -.5 * alpha - .866 * beta;

    
return

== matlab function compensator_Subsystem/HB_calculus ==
function HB  = HB_calculus(Vfaseneutro , Kh, Vcc_desired)

Vrn = Vfaseneutro(1);
Vsn = Vfaseneutro(2);
Vtn = Vfaseneutro(3);

HB = zeros(3,1);
HB(1) = Kh * ( (Vcc_desired/2)^2 - Vrn^2 );
HB(2) = Kh * ( (Vcc_desired/2)^2 - Vsn^2 );
HB(3) = Kh * ( (Vcc_desired/2)^2 - Vtn^2 );

return

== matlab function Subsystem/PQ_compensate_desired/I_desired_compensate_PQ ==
function [Ialpha , Ibeta] =   I_desired_compensate_PQ( Valpha , Vbeta , Gp , Gq)

I = [Gp Gq; -Gq Gp] * [Valpha ; Vbeta];
Ialpha = I(1);
Ibeta = I(2);


% *** Gq ***
% VaFN and VbFN depahse 90º, if one values peak, the other values 0
% Q3F = 3*.5 * ( VaFN * IbFN - VbFN * IaFN ) and VaFN_RMS = 230 Volts
% Q3F(VaFN values peak) = 3*.5((sqt(2))*230*IbFN - 0*IaFN), then: 
% IbFN(VaFN values peak) = Q3F(VaFN values peak)/(3*.5((sqt(2))*230) (1)
% Here: IbFN = -Gq * VaFN + Gp * VbFN, then
% IbFN(VaFN values peak) = -Gq(VaFN values peak) * VaFN(VaFN values peak) + Gp * VbFN(VaFN values peak)
% = -Gq(VaFN values peak) * (sqt(2))*230 + Gp * 0 (2)
% (1) and (2):
% Q3F(VaFN values peak)/(3*.5((sqt(2))*230) = -Gq(VaFN values peak) * (sqt(2))*230, then:
% Gq(VaFN values peak) = -Q3F(VaFN values peak)/(3*.5((sqt(2))*230) / ((sqt(2))*230)
%  = -Q3F(VaFN values peak)/(3*.5*2*230^2)
%

== matlab function compensator_Subsystem/measured&desired_to_SuSvSw/Embedded
MATLAB Function ==
function [Su, Sv, Sw] = sliding(Iu, Iv, Iw, Iu1, Iv1, Iw1, H)

if ( isempty(Iu) )%|| isempty(Iv) || isempty(Iw) )
    Iu = 0;
    Iv = 0;
    Iw = 0;
end

persistent pSu pSv pSw;
if ( isempty(pSu) )%|| isempty(pSv) || isempty(pSw) )
    pSu = 0;
    pSv = 0;
    pSw = 0;
end

Hu = H(1);
Hv = H(2);
Hw = H(3);

% Sliding on currents
if (Iu >= (Iu1+Hu))
    pSu = 0;
elseif (Iu < (Iu1-Hu))
    pSu = 1;
% else (Iu1 < (Iu+H)) & (Iu1 >= (Iu-H))
    % pSu mantain value cause it is 'persistent'
end

if (Iv >= (Iv1+Hv))
    pSv = 0;
elseif (Iv < (Iv1-Hv))
    pSv = 1;
end

if (Iw >= (Iw1+Hw))
    pSw = 0;
elseif (Iw < (Iw1-Hw))
    pSw = 1;
end

% Inverter state
Su = pSu;
Sv = pSv;
Sw = pSw;

% comprobar q disparo es On ó Off
% if ~(Su==0 || Su==1) % if it is NOT 0 or 1
%     error('error Su is not right')
% end
% if ~(Sv==0 || Sv==1) 
%     error('error Sv is not right')
% end
% if ~(Sw==0 || Sw==1) 
%     error('error Sw is not right')
% end

return

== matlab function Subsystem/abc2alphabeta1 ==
function [alpha, beta] = abc2alphabeta(a, b, c)

persistent k1 k2 k3;

if isempty(k1)
    k1 = 2 / 3;
end
if isempty(k2)
    k2 = 1 / 3;
end
if isempty(k3)
    k3 = sqrt(3) / 3;
end

alpha = a * k1 - b * k2 - c * k2;
beta  =          b * k3 - c * k3;
% gamma = a * k2 + b * k2 + c * k2;

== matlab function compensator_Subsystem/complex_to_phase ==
function [Vr,Vs,Vt] = complex_to_phase(Vrs,Vst,Vtr)

if ( isempty(Vrs) || isempty(Vst) || isempty(Vtr) )
    Vrs = 0;
    Vst = 0;
    Vtr = 0;
end

Vr=(Vrs-Vtr)/3;
Vs=(Vst-Vrs)/3;
Vt=(Vtr-Vst)/3;

% % Vrs=Vr-Vs
% % Vst=Vs-Vt
% % Vtr=Vt-Vr
% % Así que A*y=x=[Vr,Vs,Vt]'
% % A=[ 1 -1 0;...
% %     0 1 -1;...
% %     -1 0 1];
% % B=[Vrs Vst Vtr]';
% % NO TVENE SOLUCVÓN
% 
% 
% % Suponemos que hubVera neutro: Vr+Vs+Vt=0
% A=[ 1 -1 0;...
%     0 1 -1;...
%     1 1 1];
% B=[Vrs Vst 0]';
% 
% X=lVnsolve(A,B);% solves the linear system A*X=B
% 
% Vr=X(1);
% Vs=X(2);
% Vt=X(3);

return
